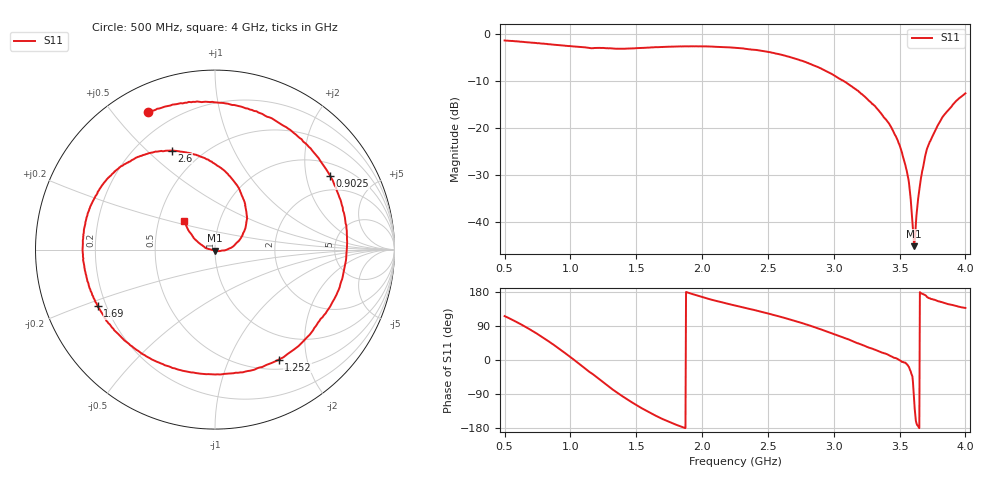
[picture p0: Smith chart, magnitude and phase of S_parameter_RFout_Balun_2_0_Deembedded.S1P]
!Agilent Technologies,E5071B,MY42403504,A.06.51
!Date: Wed Feb 26 14:54:46 2014
!Data & Calibration Information:
!Freq	S11:SOLT1(ON)
# Hz S dB R 50
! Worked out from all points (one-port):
!   801 points, 500 MHz to 4 GHz, reference 50 ohm
!   lowest |S11| = -45.1 dB at 3.611 GHz (marker M1), VSWR 1.01, Z = 49.9 - j0.54 ohm
!   |S11| at or under -10 dB: 3.074 GHz to end of sweep
!   S11 on the Smith chart (normalised r, x): 500 MHz: 0.11, +0.62; 902.5 MHz: 1.41, +2.76; 1.252 GHz: 0.63, -1.55; 1.69 GHz: 0.17, -0.22; 2.6 GHz: 0.35, +0.60; 4 GHz: 0.68, +0.23
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5e8  -1.40 115.8
6.09375e8  -1.60 96.9
7.1e8  -1.87 77.0
8.0625e8  -2.11 55.9
9.025e8  -2.37 32.7
9.375e8  -2.47 23.9
1.08625e9  -2.80 -15.5
1.2525e9  -3.00 -60.0
1.375e9  -3.16 -91.0
1.536875e9  -2.99 -126.3
1.69e9  -2.78 -154.2
1.8125e9  -2.68 -172.3
2.035625e9  -2.67 162.6
2.25e9  -2.96 143.7
2.6e9  -4.42 113.5
2.6875e9  -5.09 104.9
2.936875e9  -7.84 76.5
3.125e9  -10.96 52.5
3.4225e9  -19.18 12.2
3.50125e9  -23.74 -0.7
3.5625e9  -30.25 -13.7
3.5975e9  -39.83 -43.3
3.610625e9  -45.13 -102.5
3.62375e9  -40.43 -160.3
3.6675e9  -29.93 175.5
3.72e9  -23.59 163.6
3.83375e9  -17.39 151.3
4e9  -12.64 137.4
